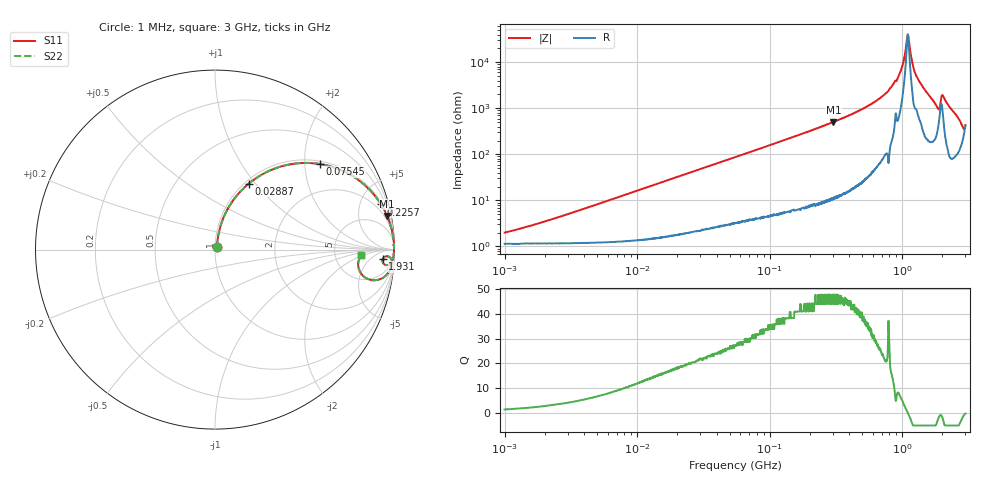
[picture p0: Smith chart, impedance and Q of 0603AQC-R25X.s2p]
!s-Parameter Generated by FASTRON Sdn. Bhd.
!FASTRON P/N : 0603AQC-R25X
!Keysight Technologies: E4991B_MY54100416_A.01.15
!Date: Thu Jun 25 14:06:54 2026
!Version  :Rev00  Thu Jun 25 14:06:54 2026
!Data & Calibration Information:
!Freq  S11  S21  S12  S22
!PortZ  Port1:50+j0  Port2:50+j0
!When reading reference impedance value at option line is always used.
! Remarks : This data is being provided solely for informational purposes.
# Hz S dB R 50
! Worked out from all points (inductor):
!   1601 points, 1 MHz to 3 GHz, reference 50 ohm
!   read as one part in series: L = 260 nH near 2.15 MHz
!   highest Q = 47.7 at 303.2 MHz (marker M1), where L = 266 nH
!   self-resonance near 1.103 GHz
!   S11 on the Smith chart (normalised r, x): 1 MHz: 1.02, +0.03; 28.87 MHz: 1.04, +0.92; 75.45 MHz: 1.08, +2.38; 225.7 MHz: 1.17, +7.31; 1.931 GHz: 18, -15; 3 GHz: 9.46, -1.78
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1000000  -34.10 54.4  -0.10 -0.9  -0.10 -0.9  -34.10 54.4
3804036  -24.10 75.7  -0.12 -3.5  -0.12 -3.5  -24.10 75.7
1.447069e7  -13.00 73.3  -0.36 -13.0  -0.36 -13.0  -13.00 73.3
2.886629e7  -7.69 63.0  -1.00 -24.3  -1.00 -24.3  -7.69 63.0
5.504702e7  -3.80 47.7  -2.62 -40.2  -2.62 -40.2  -3.80 47.7
7.544761e7  -2.45 39.2  -3.98 -48.9  -3.98 -48.9  -2.45 39.2
2.083556e8  -0.42 16.5  -10.90 -72.2  -10.90 -72.2  -0.42 16.5
2.257233e8  -0.36 15.2  -11.60 -73.5  -11.60 -73.5  -0.36 15.2
3.032461e8  -0.20 11.1  -14.30 -77.6  -14.30 -77.6  -0.20 11.1
5.63991e8  -0.05 4.9  -21.40 -83.4  -21.40 -83.4  -0.05 4.9
7.925923e8  -0.02 2.3  -27.90 -86.0  -27.90 -86.0  -0.02 2.3
9.490412e8  -0.02 1.1  -34.50 -81.5  -34.50 -81.5  -0.02 1.1
1.01283e9  -0.02 0.6  -39.30 -76.3  -39.30 -76.3  -0.02 0.6
1.080907e9  -0.02 0.1  -48.90 -45.4  -48.90 -45.4  -0.02 0.1
1.108292e9  -0.02 -0.0  -51.90 11.1  -51.90 11.1  -0.02 -0.0
1.218836e9  -0.02 -0.8  -37.50 79.6  -37.50 79.6  -0.02 -0.8
1.307284e9  -0.03 -1.2  -33.10 79.1  -33.10 79.1  -0.03 -1.2
1.827992e9  -0.23 -5.0  -21.00 70.3  -21.00 70.3  -0.23 -5.0
1.931433e9  -0.57 -3.2  -21.60 38.4  -21.60 38.4  -0.57 -3.2
2.050964e9  -0.15 -3.0  -25.20 70.0  -25.20 70.0  -0.15 -3.0
2.769173e9  -0.66 -10.4  -14.40 62.2  -14.40 62.2  -0.66 -10.4
3e9  -1.78 -2.2  -14.50 9.6  -14.50 9.6  -1.78 -2.2
